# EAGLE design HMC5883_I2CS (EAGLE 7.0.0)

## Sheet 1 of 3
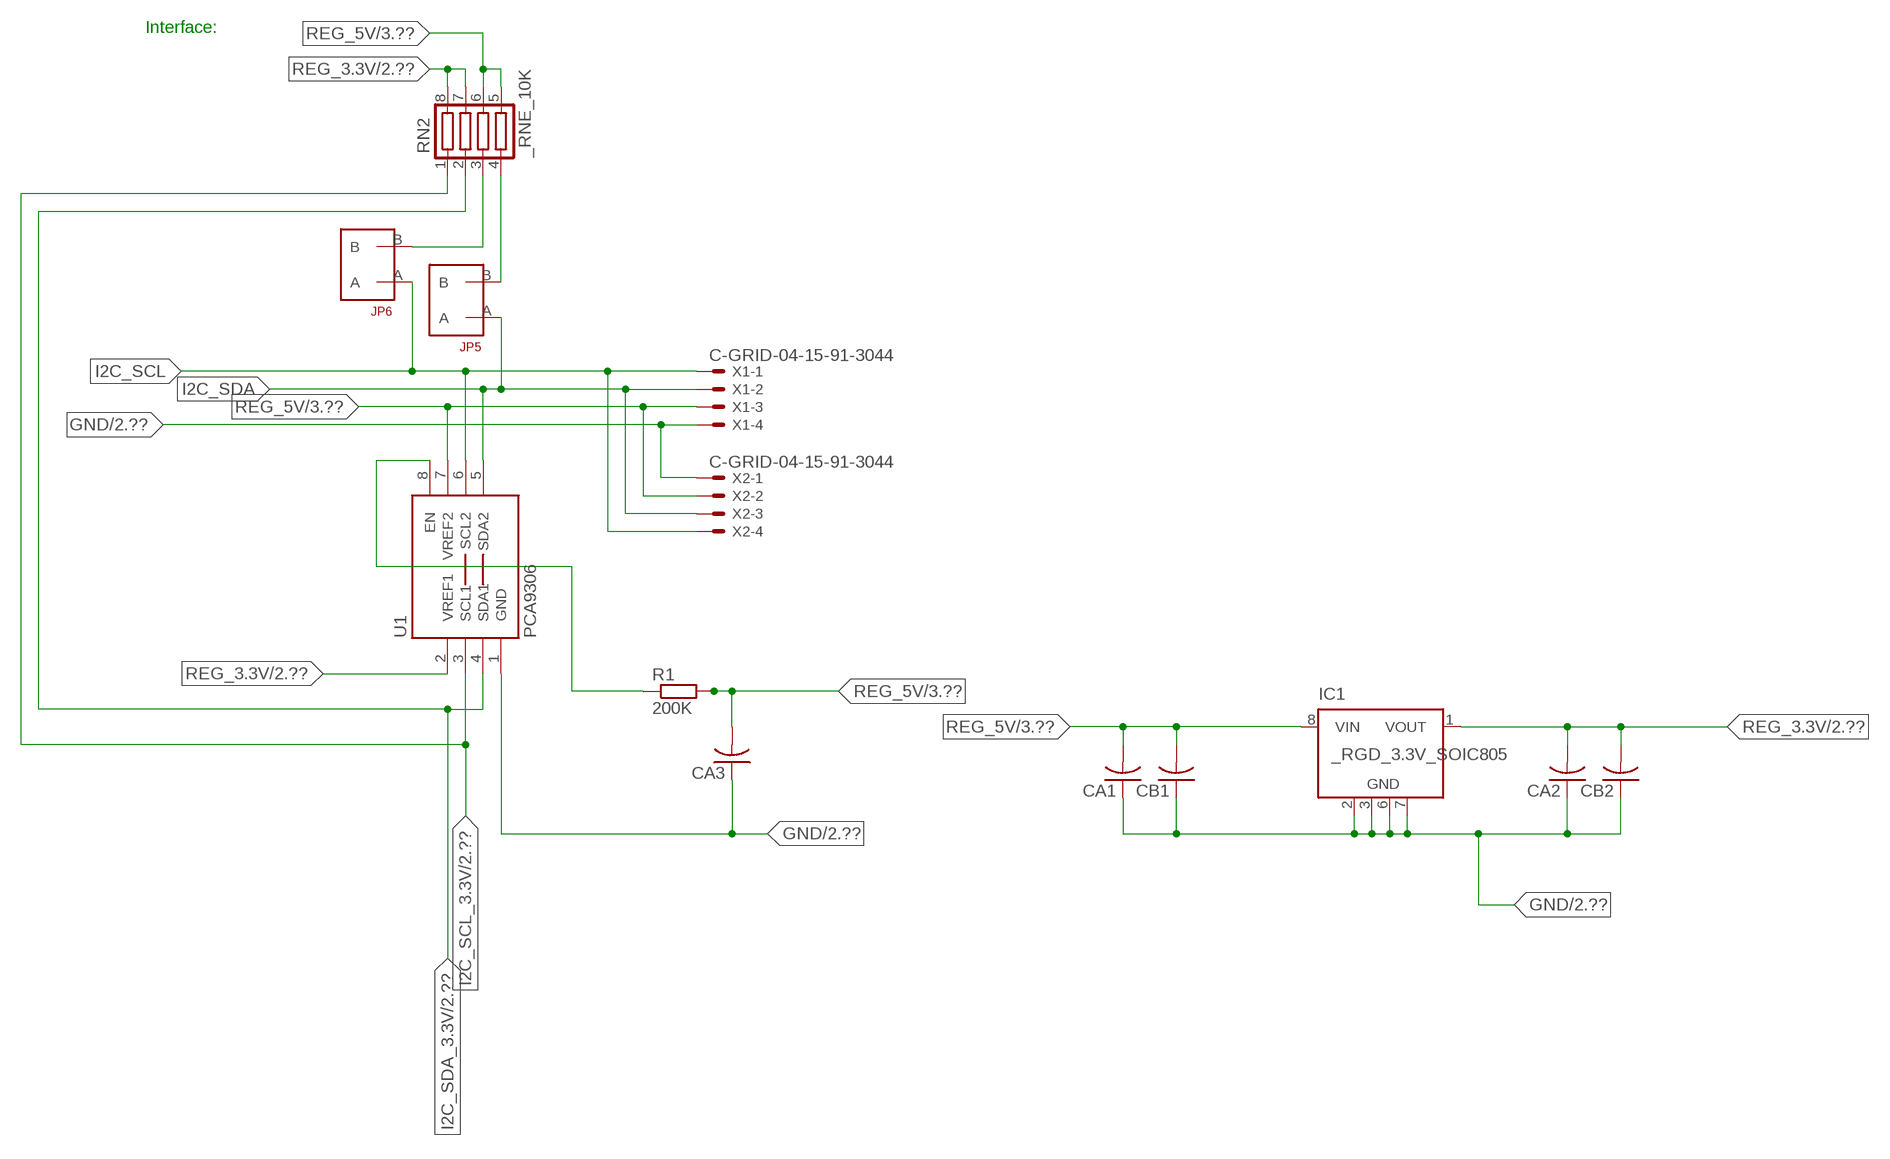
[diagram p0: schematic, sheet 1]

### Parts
CA1  CC1206KRX7R9BB104  [.1UF]
CA2  CC1206KRX7R9BB104  [.1UF]
CA3  CC1206KRX7R9BB104  [.1UF]
CB1  TMK316F106ZL-TC1206K  [TMK316F106ZL-T]
CB2  TMK316F106ZL-TC1206K  [TMK316F106ZL-T]
IC1  _RGD_3.3V_SOIC805  [_RGC_3.3V_SOIC8]
JP5  JUMPER_1X2_2MM  [JUMPER_1X2_2MM]
JP6  JUMPER_1X2_2MM  [JUMPER_1X2_2MM]
R1  200K  RESISTOR_SMT-0603  [R603]
RN2  _RNE_10K  [RNE]
U1  PCA9306  PCA9306_NCD  [PSOP-8]
X1  C-GRID-04-15-91-3044  [15-91-04]
X2  C-GRID-04-15-91-3044  [15-91-04]

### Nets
GND: CA1.1 CA2.1 CA3.1 CB1.1 CB2.1 IC1.2(GND) IC1.3(GND) IC1.6(GND) IC1.7(GND) U1.1(GND) X1.4 X2.1 ; also sheet 2,3
I2C_SCL: JP6.A U1.6(SCL2) X1.1 X2.4
I2C_SCL_3.3V: RN2.1 U1.3(SCL1) ; also sheet 2
I2C_SDA: JP5.A U1.5(SDA2) X1.2 X2.3
I2C_SDA_3.3V: RN2.2 U1.4(SDA1) ; also sheet 2
N$1: JP6.B RN2.3
N$2: JP5.B RN2.4
N$26: R1.1 U1.8(EN)
REG_3.3V: CA2.2 CB2.2 IC1.1(VOUT) RN2.7 RN2.8 U1.2(VREF1) ; also sheet 2
REG_5V: CA1.2 CA3.2 CB1.2 IC1.8(VIN) R1.2 RN2.5 RN2.6 U1.7(VREF2) X1.3 X2.2 ; also sheet 3
Unconnected: IC1.4(NC) IC1.5(NC)

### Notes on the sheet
- Interface:

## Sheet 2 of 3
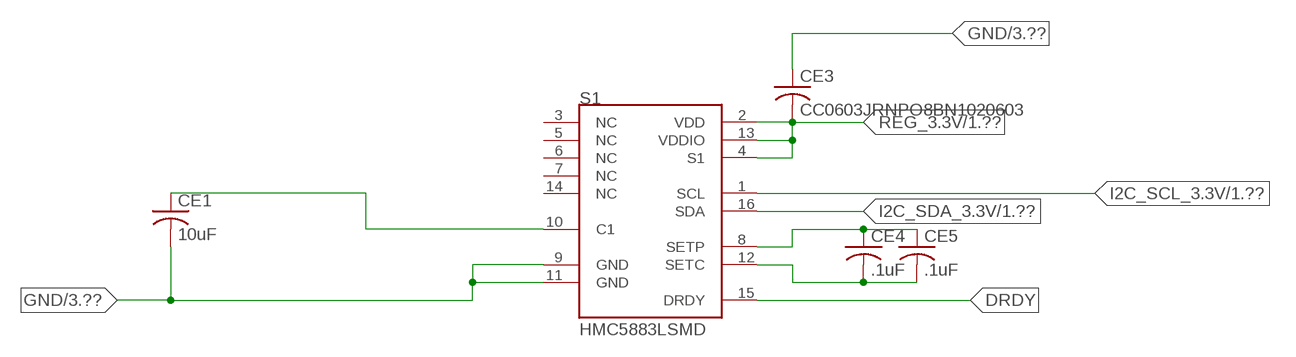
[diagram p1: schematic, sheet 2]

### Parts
CE1  10uF  _CB_10UF_25VC1206K  [_CB_10UF_25V]
CE3  CC0603JRNPO8BN1020603  [CC0603JRNPO8BN102]
CE4  .1uF  CC0603JRNPO8BN1020603  [CC0603JRNPO8BN102]
CE5  .1uF  CC0603JRNPO8BN1020603  [CC0603JRNPO8BN102]
S1  HMC5883LSMD  [16LPCC]

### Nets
DRDY: S1.15(DRDY)
GND: CE1.2 CE3.1 S1.9(GND) S1.11(GND) ; also sheet 1,3
I2C_SCL_3.3V: S1.1(SCL) ; also sheet 1
I2C_SDA_3.3V: S1.16(SDA) ; also sheet 1
N$4: CE1.1 S1.10(C1)
N$7: CE4.1 CE5.1 S1.8(SETP)
N$8: CE4.2 CE5.2 S1.12(SETC)
REG_3.3V: CE3.2 S1.2(VDD) S1.4(S1) S1.13(VDDIO) ; also sheet 1
Unconnected: S1.3(NC) S1.5(NC) S1.6(NC) S1.7(NC) S1.14(NC)

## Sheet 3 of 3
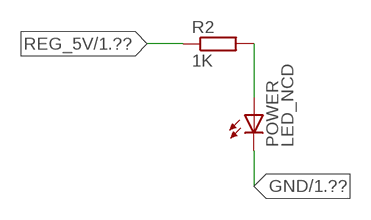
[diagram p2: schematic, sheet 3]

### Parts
POWER  LED_NCD  [CHIPLED_0603]
R2  1K  RESISTOR_SMT-0402  [R402]

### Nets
GND: POWER.C ; also sheet 1,2
N$5: POWER.A R2.2
REG_5V: R2.1 ; also sheet 1

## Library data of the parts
CA1-CA3 = NCD_ULTIMATE_LIBRARY:CC1206KRX7R9BB104: Capacitor CA .1uF 50V SMT C1206K CC1206KRX7R9BB104
CB1 CB2 = NCD_ULTIMATE_LIBRARY:TMK316F106ZL-T: Capacitor CB 10uF SMT 1206 TMK316F106ZL-T
CE1 = NCD_ULTIMATE_LIBRARY:_CB_10UF_25V: Capacitor 10uF SMT
CE3-CE5 = NCD_ULTIMATE_LIBRARY:CC0603JRNPO8BN102: Capacitor CE 1uF SMT CC0603JRNPO8BN102 0603
IC1 = NCD_ULTIMATE_LIBRARY:_RGD_3.3V_SOIC8: Regulator Linear 3.3V Chip Positive VOLTAGE REGULATOR Digikey 497-1199-2-ND/L78L33ACD13TR
JP5 JP6 = NCD_ULTIMATE_CONNECTORS:JUMPER_1X2_2MM
POWER = NCD_ULTIMATE_LIBRARY:LED_NCD: LED Digikey 754-1132-2-ND/APT2012SRCPRV
R1 R2 = NCD_ULTIMATE_LIBRARY:RESISTOR_SMT: NCD Resistor
RN2 = NCD_ULTIMATE_LIBRARY:_RNE_10K: Resistor Array RNE SMT 10K x 4 Single Resistor Source: http://www.ctscorp.com/components/Datasheets/CTSChipArrayDs.pdf Digikey 742C083103JPTR-ND/742C083103JP; OC_FARNELL: unknown; OC_NEWARK: unknown
S1 = NCD_ULTIMATE_bhaskar:HMC5883L: 3 Axis Digital Compass IC Digikey 342-1082-2-ND/HMC5883L-TR
U1 = NCD_ULTIMATE_LIBRARY:PCA9306_NCD: NCD Bidirectional I2C level shifter. NOT compatible with all available part number pinout schemes- DOUBLE CHECK!!!; PROD_ID: IC-10023
X1 X2 = NCD_ULTIMATE_CONNECTORS:C-GRID-04: CONNECTOR 4-Pos I2C wire to board 2.54 mm (0.100") pitch header Digikey WM1342-ND/0015912045; OC_FARNELL: unknown; OC_NEWARK: unknown

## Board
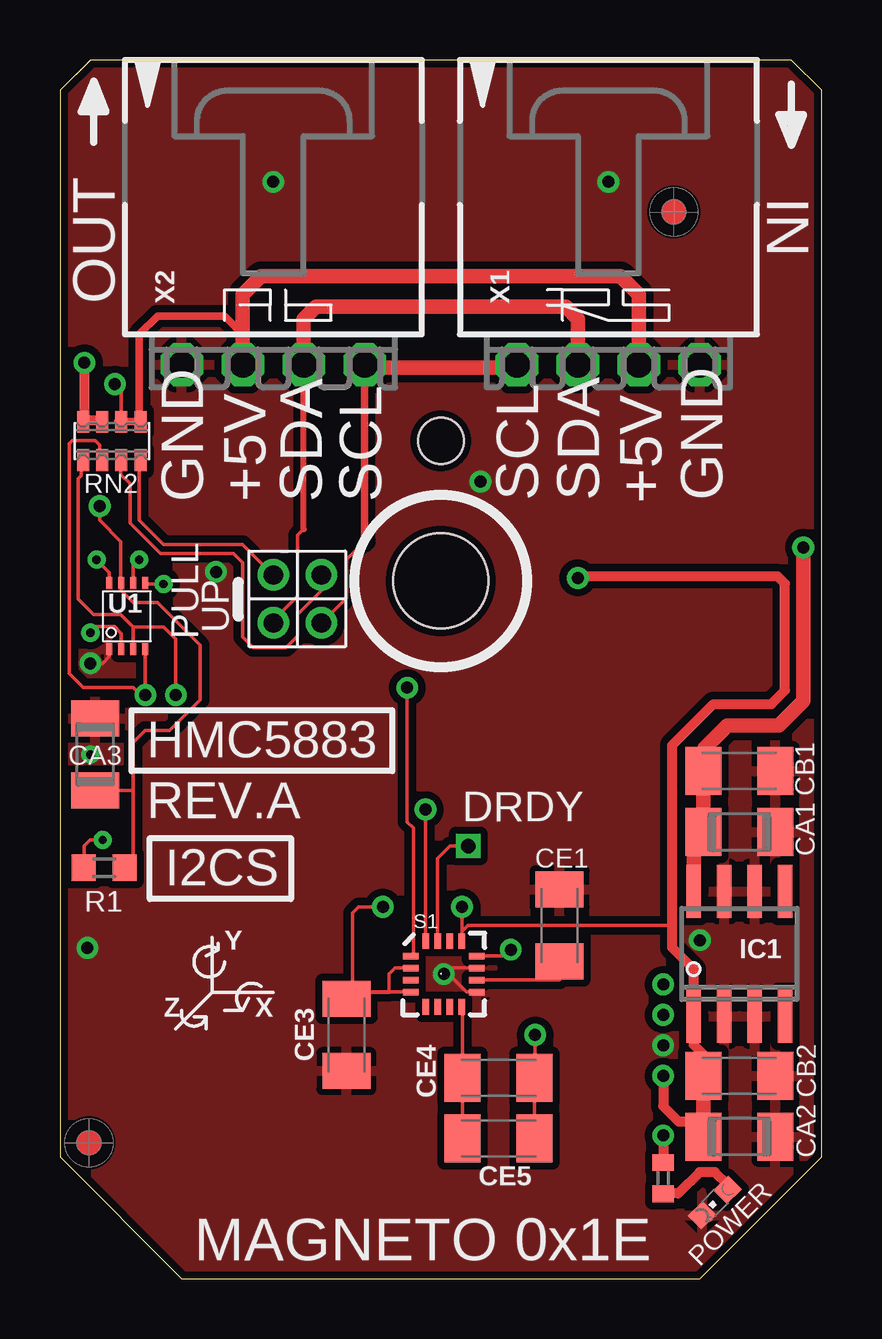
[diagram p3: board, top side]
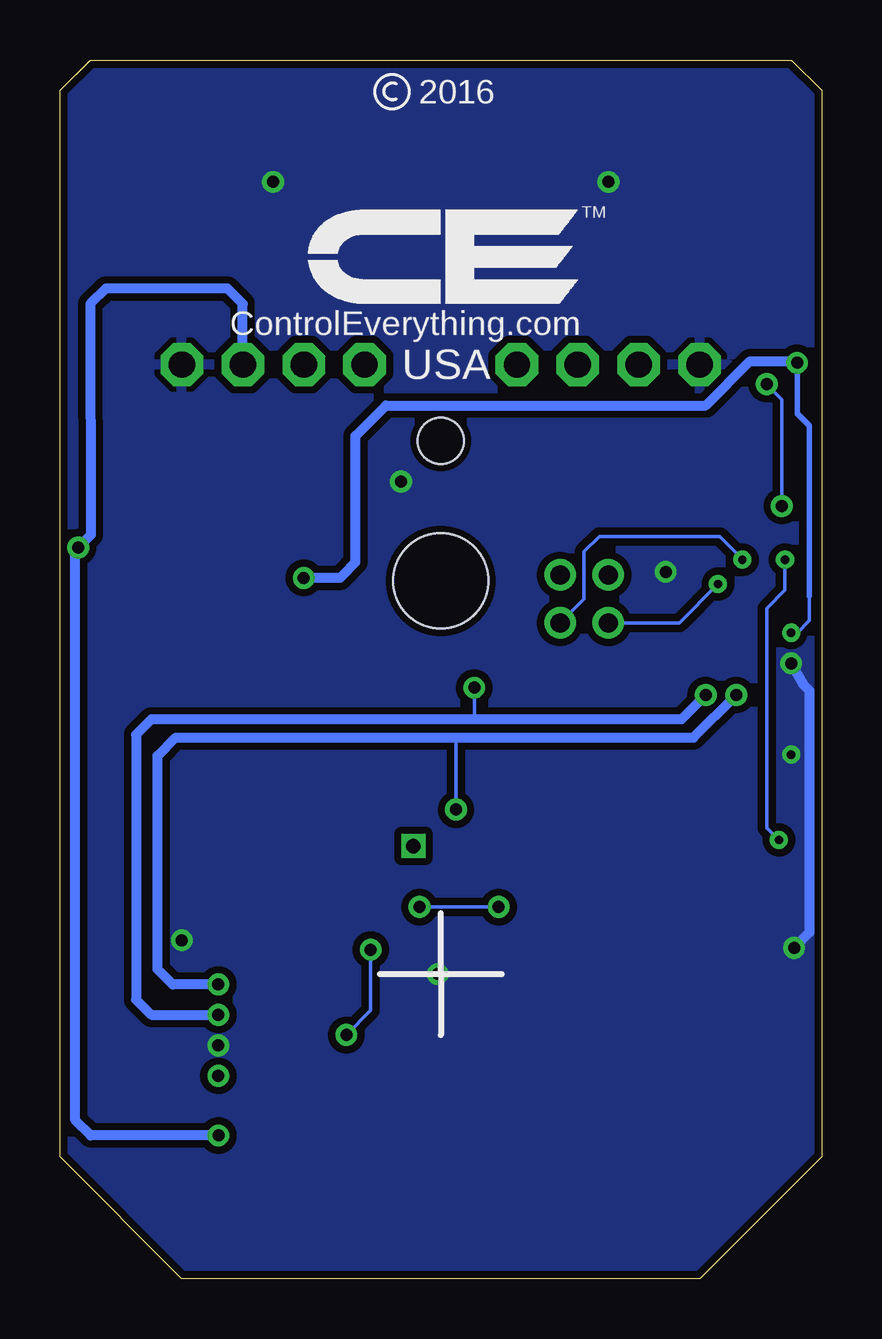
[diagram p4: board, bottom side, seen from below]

Size 31.75 x 50.8 mm. Coordinates in mm from the lower left corner, seen from the top.
Outline: 48 segments
Copper layers (1*16): Top 0.035mm / dielectric 1.5mm / Bottom 0.035mm
Design rules "default": minimum track width 5mil, minimum drill 24mil, track to track 5mil, track to pad 5mil, pad to pad 5mil, via to via 5mil, smd to smd 5mil, copper to edge 10mil, drill to drill 8mil, minimum pad ring 10mil, minimum via ring 8mil, stop-mask expansion 2mil, vias tented up to drill 0mil, thermal gap 10mil
Holes 3.96 mm at 15.88,29.08
Holes 1.91 mm at 15.88,34.93

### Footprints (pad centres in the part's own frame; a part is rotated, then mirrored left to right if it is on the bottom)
.1UF = smd 1.5 x 2: 1 -1.5,0; 2 1.5,0
TMK316F106ZL-T = smd 1.5 x 2: 1 -1.5,0; 2 1.5,0
_CB_10UF_25V = smd 1.5 x 2: 1 -1.5,0; 2 1.5,0
CC0603JRNPO8BN102 = smd 1.5 x 2: 1 -1.5,0; 2 1.5,0
_RGC_3.3V_SOIC8 = smd 0.6 x 2.2: 1 -1.905,-2.6; 2 -0.635,-2.6; 3 0.635,-2.6; 4 1.905,-2.6; 5 1.905,2.6; 6 0.635,2.6; 7 -0.635,2.6; 8 -1.905,2.6
JUMPER_1X2_2MM = drill 0.8: A 0,2; B 0,0
CHIPLED_0603 = smd 0.8 x 0.876: A 0,-0.75; C 0,0.75
R603 = smd 1 x 1.1: 1 -0.85,0; 2 0.85,0
R402 = smd 0.7 x 0.9: 1 -0.65,0; 2 0.65,0
RNE = smd 0.5 x 0.9: 1 -1.2,-0.8; 2 -0.4,-0.8; 3 0.4,-0.8; 4 1.2,-0.8; 5 1.2,0.8; 6 0.4,0.8; 7 -0.4,0.8; 8 -1.2,0.8
16LPCC = smd 0.65 x 0.28: 1 -1.37,0.75; 2 -1.37,0.25; 3 -1.37,-0.25; 4 -1.37,-0.75; 9 1.37,-0.75; 10 1.37,-0.25; 11 1.37,0.25; 12 1.37,0.75 | smd 0.28 x 0.65: 5 -0.75,-1.37; 6 -0.25,-1.37; 7 0.25,-1.37; 8 0.75,-1.37; 13 0.75,1.37; 14 0.25,1.37; 15 -0.25,1.37; 16 -0.75,1.37
PSOP-8 = smd 0.25 x 0.5: 1 -0.73,-1.37; 2 -0.23,-1.37; 3 0.27,-1.37; 4 0.77,-1.37; 5 0.77,1.38; 6 0.27,1.38; 7 -0.23,1.38; 8 -0.73,1.38
15-91-04 = drill 1.1 pad 1.778 octagon: 1 -3.81,-7.62; 2 -1.27,-7.62; 3 1.27,-7.62; 4 3.81,-7.62

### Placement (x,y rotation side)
CA1  28.32,18.62 180 top
CA2  28.32,5.92 180 top
CA3  1.46,21.86 270 top
CB1  28.32,21.16 180 top
CB2  28.32,8.46 180 top
CE1  20.83,14.73 90 top
CE3  11.94,10.16 90 top
CE4  18.29,8.38 0 top
CE5  18.29,5.84 0 top
IC1  28.32,13.54 0 top
JP5  8.89,29.34 180 top
JP6  10.9,29.34 180 top
POWER  27.3,3.18 135 top
R1  1.84,17.13 0 top
R2  25.15,4.19 270 top
RN2  2.16,34.93 0 top
S1  16,12.7 0 top
U1  2.79,27.61 0 top
U$5  [VISION_REF10]  1.21,5.66 90 top
U$28  [VISION_REF10]  25.59,44.46 90 top
X1  22.86,45.72 0 top
X2  8.89,45.72 0 top

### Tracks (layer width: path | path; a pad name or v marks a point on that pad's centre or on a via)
DRDY  (via drill 0.6)
  Top 0.152: S1.15 15.75,17.53 16.26,18.03 v17.02,18.03
GND  (via drill 0.35, 0.5)
  Top 0.152: CA3.1 1.52,23.42 1.52,23.62 | S1.11 16.76,12.95 16,12.95 v16,12.7 16.2,12.7 16.94,11.96 17.36,11.96 S1.9 | v1.27,25.65 1.78,25.65 2.06,25.94 U1.1
  Bottom 0.406: v1.27,25.65 0.76,24.77 0.51,24.51 0.51,14.43 v1.15,13.79
  other vias: 8.89,45.72 22.86,45.72 25.15,9.73 17.53,33.22 26.67,14.11 6.5,29.46 1.27,21.84
  pour Bottom (isolate 0.305): -0.64,5.08 -0.64,49.53 1.27,51.44 30.48,51.44 32.38,49.53 32.38,5.08 26.67,-0.63 5.08,-0.63
  pour Top (isolate 0.305): 4.45,-1.27 -1.27,4.45 -1.27,50.17 0.64,52.07 31.11,52.07 33.02,50.17 33.02,4.45 27.3,-1.27
I2C_SCL  (via drill 0.35)
  Top 0.152: 12.7,30.73 11.94,29.97 11.94,28.38 JP6.A | v3.3,29.97 3.06,29.73 U1.6
  Top 0.305: 12.7,30.73 X2.4
  Top 0.406: X2.4 12.7,37.97 | 19.05,37.97 X1.1
  Top 0.61: 12.7,37.97 19.05,37.97
  Bottom 0.152: JP6.A 9.91,28.33 9.91,30.3 9.27,30.94 4.24,30.94 3.3,30 v3.3,29.97
I2C_SCL_3.3V  (via drill 0.5)
  Top 0.152: RN2.1 0.89,34.07 0.89,33.48 0.77,33.35 0.77,28.33 1.41,27.69 2.54,27.69 3.06,27.17 | S1.1 14.73,13.55 14.73,18.8 14.48,19.05 v14.48,24.64 | 3.06,27.17 U1.3 | v4.83,24.33 v4.83,24.34 4.83,26.67 4.33,27.17 3.06,27.17
  Bottom 0.152: v14.48,24.64 14.48,23.32
  Bottom 0.406: v4.83,24.33 5.84,23.32 14.48,23.32 27.94,23.32 28.58,22.68 28.58,11.63 27.94,11 v25.15,11
I2C_SDA  (via drill 0.35)
  Top 0.152: JP5.A 8.89,27.44 9.91,28.45 9.91,30.99 10.16,31.24 | U1.5 3.6,28.96 v4.32,28.96
  Top 0.254: 10.16,31.24 10.16,31.25 X2.3
  Top 0.61: X2.3 10.16,40.01 10.67,40.51 21.09,40.51 21.59,40.01 X1.2
  Bottom 0.152: v4.32,28.96 5.94,27.34 JP5.A
I2C_SDA_3.3V  (via drill 0.5)
  Top 0.152: RN2.2 1.65,34.14 1.65,34.75 1.46,34.94 0.51,34.94 0.38,34.81 0.38,26.37 0.38,26.36 0.38,25.22 0.96,24.64 3.05,24.64 3.35,24.33 v3.56,24.33 v3.56,24.34 U1.4 | S1.16 15.24,14.06 | 15.24,14.06 15.24,13.97 | 15.24,14.06 v15.24,19.56
  Bottom 0.152: v15.24,19.56 15.24,22.56
  Bottom 0.406: v25.15,12.27 27.05,12.27 27.69,12.9 27.69,21.79 26.93,22.56 15.24,22.56 5.34,22.56 v3.56,24.33
N$1
  Top 0.152: JP6.B 10.92,29.31 10.92,28.7 9.91,27.69 9.91,26.8 9.42,26.31 8.06,26.31 7.62,26.75 7.62,29.84 7.24,30.23 4.19,30.23 2.92,31.5 2.92,33.15 2.54,33.53 2.54,34.1 RN2.3
  Top 0.305: 2.54,34.02 RN2.3
N$2
  Top 0.152: JP5.B 7.62,30.61 4.32,30.61 3.3,31.62 3.3,34.07 RN2.4
  Top 0.305: 3.37,33.88 RN2.4
N$4
  Top 0.152: S1.10 20.83,12.45 CE1.1
N$5
  Top 0.406: POWER.A 27.84,3.92 27.3,4.45 26.67,4.45 25.78,3.56 25.16,3.56 R2.2
N$7
  Top 0.152: S1.8 16.79,11.29 CE4.1 CE5.1
N$8  (via drill 0.5)
  Top 0.152: CE5.2 CE4.2 19.81,8.41 v19.81,10.16 | v18.8,13.72 18.53,13.45 S1.12
  Bottom 0.152: v19.81,10.16 18.8,11.18 v18.8,13.72
N$26  (via drill 0.35)
  Top 0.152: R1.1 1.02,17.16 1.02,18.03 1.27,18.29 v1.78,18.29 | v1.52,29.97 2.06,29.44 U1.8
  Bottom 0.152: v1.78,18.29 2.29,18.8 2.29,27.94 1.52,28.7 v1.52,29.97
REG_3.3V  (via drill 0.35, 0.5)
  Top 0.152: CE3.2 12.23,11.95 13.72,11.95 | 13.72,11.95 S1.4 | 13.72,11.95 13.72,12.7 13.97,12.95 S1.2 | 16.76,14.48 16.76,14.08 S1.13 | 16.76,14.48 17.02,14.73 25.53,14.73 | 16.76,14.48 v16.76,15.49 | 13.72,11.95 13.72,11.94 12.19,11.94 12.19,15.24 12.45,15.49 v13.46,15.49 | v1.27,26.92 1.52,27.18 2.29,27.18 2.56,26.9 U1.2
  Top 0.406: CB2.2 26.82,9.35 26.42,9.75 26.42,10.36 | v25.15,8.46 25.15,7.19 25.78,6.55 26.82,6.55 | IC1.1 26.42,12.9 25.53,13.79 25.53,14.73 25.53,22.24 27.24,23.95 29.66,23.95 30.23,24.52 30.23,28.97 29.91,29.29 21.67,29.29 v21.59,29.21 | 26.52,5.62 CA2.2 | v1.02,38.18 1.02,35.78 | 1.02,35.78 RN2.8 | 1.02,35.78 1.71,35.78 RN2.7
  Top 0.61: CB2.2 26.82,6.55 CA2.2 | 26.42,10.36 IC1.1
  Bottom 0.152: v16.76,15.49 v13.46,15.49 | 0.51,28.45 0.51,27.43 1.02,26.92 v1.27,26.92
  Bottom 0.229: 0.51,28.45 0.51,35.56 1.02,36.07 v1.02,38.18
  Bottom 0.406: v1.02,38.18 1.08,38.24 2.99,38.24 4.83,36.4 18.16,36.4 19.43,35.13 19.43,29.87 19.94,29.34 20.07,29.21 v21.59,29.21
REG_5V  (via drill 0.5)
  Top 0.152: RN2.6 2.56,37.01 v2.29,37.29 | R1.2 3.05,17.49 3.05,20.36 | 3.05,20.36 3.05,22.35 3.56,22.86 4.57,22.86 5.84,24.13 5.84,26.42 4.06,28.19 3.05,28.19 2.56,28.68 U1.7 2.54,29.01 2.54,30.73 1.65,31.62 v1.65,32.21 | CA3.2 3.05,20.36
  Top 0.305: 7.62,39.37 7.5,39.37 | 2.42,35.74 RN2.6 RN2.5 3.31,35.8 3.31,39.37 4.07,40.13 6.86,40.13 7.62,39.37 | X2.2 7.62,39.37
  Top 0.406: v25.15,5.97 R2.1
  Top 0.61: X2.2 7.62,41.02 8.38,41.78 23.37,41.78 24.13,41.02 24.13,38.23 X1.3 | IC1.8 26.42,18.21 CA1.2 CB1.2 26.86,21.2 26.86,22.11 27.82,23.06 29.98,23.06 30.99,24.08 v30.99,30.48
  Bottom 0.152: v1.65,32.21 1.65,36.65 v2.29,37.29
  Bottom 0.406: X1.3 24.13,40.64 24.77,41.28 29.84,41.28 30.48,40.64 30.47,31 v30.99,30.48 31.11,30.36 31.11,6.6 30.48,5.97 v25.15,5.97

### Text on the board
tPlace: Y | Z | X | MAGNETO 0x1E
tNames: IN | OUT | GND | +5V | SDA | SCL | SCL | SDA | +5V | GND | PULL | UP | HMC5883 | REV.A | DRDY | I2CS
bNames: 2016 | TM | ControlEverything.com | USA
